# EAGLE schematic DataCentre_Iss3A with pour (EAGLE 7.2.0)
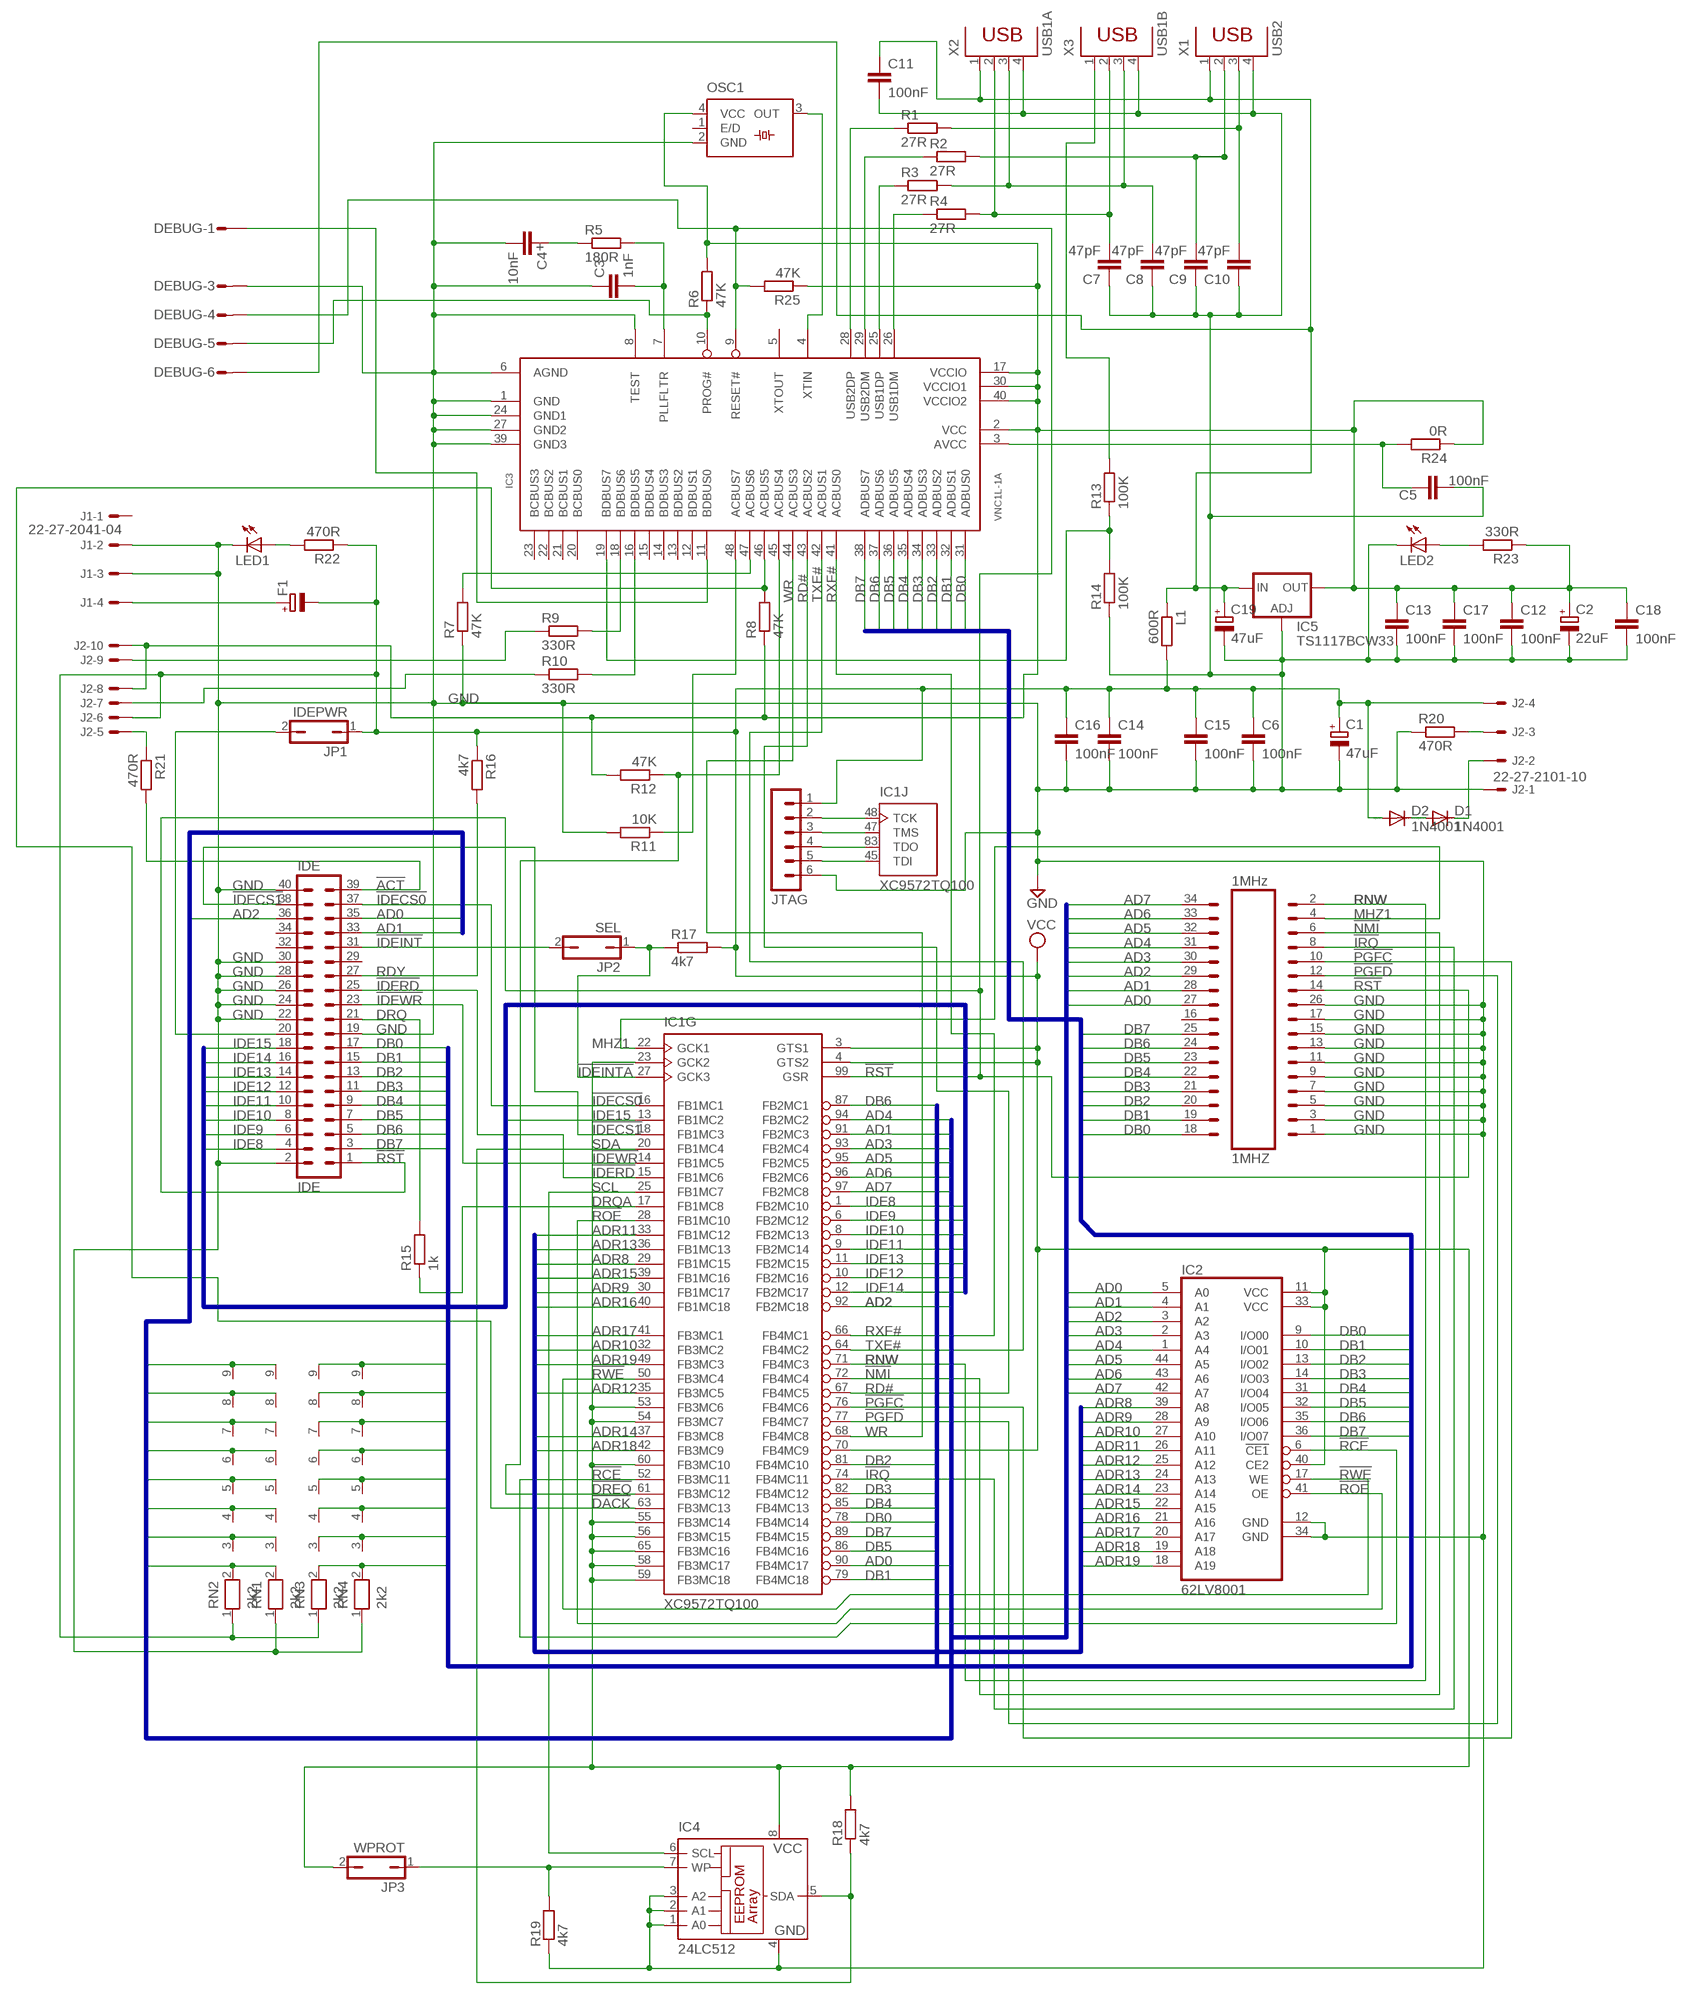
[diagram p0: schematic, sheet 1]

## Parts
C1  47uF  CPOL-EUC  [PANASONIC_C]
C2  22uF  CPOL-EUB  [PANASONIC_B]
C3  1nF  C-EUC1206K  [C1206K]
C4  10nF  C-EUC1206K  [C1206K]
C5  100nF  C-EUC1206K  [C1206K]
C6  100nF  C-EUC1206K  [C1206K]
C7  47pF  C-EUC0603K  [C0603K]
C8  47pF  C-EUC0603K  [C0603K]
C9  47pF  C-EUC0603K  [C0603K]
C10  47pF  C-EUC0603K  [C0603K]
C11  100nF  C-EUC1206K  [C1206K]
C12  100nF  C-EUC1206K  [C1206K]
C13  100nF  C-EUC1206K  [C1206K]
C14  100nF  C-EUC1206K  [C1206K]
C15  100nF  C-EUC1206K  [C1206K]
C16  100nF  C-EUC1206K  [C1206K]
C17  100nF  C-EUC1206K  [C1206K]
C18  100nF  C-EUC0603K  [C0603K]
C19  47uF  CPOL-EUC  [PANASONIC_C]
D1  1N4001  DIODE-DO35-10  [DO35-10]
D2  1N4001  DIODE-DO35-10  [DO35-10]
DEBUG  DF3-06P  [DF3P-06]
F1  CPOL-EU085CS-1R  [085CS_1R]
IC1  XC9572TQ100  [TQ100]
IC2  62LV8001  [TSOPII-Z44]
IC3  VNC1L-1A  [LQFP48]
IC4  24LC512  24LC256SN  [SO-08]
IC5  TS1117BCW33  LD117AS33TR  [SOT223]
IDE  IDE  ML40  [ML40]
J1  22-27-2041-04  [6410-04]
J2  22-27-2101-10  [6410-10]
JP1  IDEPWR  JP1Q  [JP1]
JP2  SEL  JP1Q  [JP1]
JP3  WPROT  JP1Q  [JP1]
JTAG  MA06-1  [MA06-1]
L1  600R  R-EU_R1206  [R1206]
LED1  LEDCHIPLED_0603  [CHIPLED_0603]
LED2  LEDCHIPLED_0603  [CHIPLED_0603]
OSC1  SM77HCSX750  [XTAL-CSX750]
PL1  1MHZ  [ML34]
R1  27R  R-EU_R0603  [R0603]
R2  27R  R-EU_R0603  [R0603]
R3  27R  R-EU_R0603  [R0603]
R4  27R  R-EU_R0603  [R0603]
R5  180R  R-EU_R0603  [R0603]
R6  47K  R-EU_R0603  [R0603]
R7  47K  R-EU_R0603  [R0603]
R8  47K  R-EU_R0603  [R0603]
R9  330R  R-EU_R0603  [R0603]
R10  330R  R-EU_R0603  [R0603]
R11  10K  R-EU_R0603  [R0603]
R12  47K  R-EU_R0603  [R0603]
R13  100K  R-EU_R0603  [R0603]
R14  100K  R-EU_R0603  [R0603]
R15  1k  R-EU_R0603  [R0603]
R16  4k7  R-EU_R0603  [R0603]
R17  4k7  R-EU_R0603  [R0603]
R18  4k7  R-EU_R0603  [R0603]
R19  4k7  R-EU_R0603  [R0603]
R20  470R  R-EU_R0603  [R0603]
R21  470R  R-EU_R0603  [R0603]
R22  470R  R-EU_R0603  [R0603]
R23  330R  R-EU_R0603  [R0603]
R24  0R  R-EU_R0603  [R0603]
R25  47K  R-EU_R0603  [R0603]
RN1  2k2  RN08  [RN-9]
RN2  2k2  RN08  [RN-9]
RN3  2k2  RN08  [RN-9]
RN4  2k2  RN08  [RN-9]
X1  USB2  PN87520  [PN87520]
X2  USB1A  PN87520  [PN87520]
X3  USB1B  PN61729  [PN61729]

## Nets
!ACT: IDE.39 R21.2
!DACK: IC1.63(G:FB3MC13) IC3.46(ACBUS5) R8.2
!DREQ: IC1.61(G:FB3MC12) IC3.45(ACBUS4) R12.1
!IDECS0: IC1.16(G:FB1MC1) IDE.37
!IDECS1: IC1.18(G:FB1MC3) IDE.38
!IDEINT: IDE.31 JP2.2
!IDEINTA: IC1.27(G:GCK3) JP2.1 R17.1
!IDERD: IC1.15(G:FB1MC6) IDE.25
!IDEWR: IC1.14(G:FB1MC5) IDE.23
!IRQ: IC1.74(G:FB4MC11) PL1.8(8_IRQ)
!NMI: IC1.72(G:FB4MC4) PL1.6(6_NMI)
!PGFC: IC1.76(G:FB4MC6) PL1.10(10_FC)
!PGFD: IC1.77(G:FB4MC7) PL1.12(12_FD)
!RCE: IC1.52(G:FB3MC11) IC2.6(!CE1)
!ROE: IC1.28(G:FB1MC10) IC2.41(OE)
!RST: DEBUG.4 IC1.99(G:GSR) IC3.9(RESET#) IDE.1 PL1.14(14_RST) R25.2
!RWE: IC1.50(G:FB3MC4) IC2.17(WE)
AD0: IC1.90(G:FB4MC17) IC2.5(A0) IDE.35 PL1.27(27_A0) RN1.2 RN2.2
AD1: IC1.91(G:FB2MC3) IC2.4(A1) IDE.33 PL1.28(28_A1) RN1.3 RN2.3
AD2: IC1.92(G:FB2MC18) IC2.3(A2) IDE.36 PL1.29(29_A2) RN1.4 RN2.4
AD3: IC1.93(G:FB2MC4) IC2.2(A3) PL1.30(30_A3) RN1.5 RN2.5
AD4: IC1.94(G:FB2MC2) IC2.1(A4) PL1.31(31_A4) RN1.6 RN2.6
AD5: IC1.95(G:FB2MC5) IC2.44(A5) PL1.32(32_A5) RN1.7 RN2.7
AD6: IC1.96(G:FB2MC6) IC2.43(A6) PL1.33(33_A6) RN1.8 RN2.8
AD7: IC1.97(G:FB2MC8) IC2.42(A7) PL1.34(34_A7) RN1.9 RN2.9
ADR8: IC1.29(G:FB1MC15) IC2.39(A8)
ADR9: IC1.30(G:FB1MC17) IC2.28(A9)
ADR10: IC1.32(G:FB3MC2) IC2.27(A10)
ADR11: IC1.33(G:FB1MC12) IC2.26(A11)
ADR12: IC1.35(G:FB3MC5) IC2.25(A12)
ADR13: IC1.36(G:FB1MC13) IC2.24(A13)
ADR14: IC1.37(G:FB3MC8) IC2.23(A14)
ADR15: IC1.39(G:FB1MC16) IC2.22(A15)
ADR16: IC1.40(G:FB1MC18) IC2.21(A16)
ADR17: IC1.41(G:FB3MC1) IC2.20(A17)
ADR18: IC1.42(G:FB3MC9) IC2.19(A18)
ADR19: IC1.49(G:FB3MC3) IC2.18(A19)
DB0: IC1.78(G:FB4MC14) IC2.9(I/O00) IC3.31(ADBUS0) IDE.17 PL1.18(18_D0) RN3.2 RN4.2
DB1: IC1.79(G:FB4MC18) IC2.10(I/O01) IC3.32(ADBUS1) IDE.15 PL1.19(19_D1) RN3.3 RN4.3
DB2: IC1.81(G:FB4MC10) IC2.13(I/O02) IC3.33(ADBUS2) IDE.13 PL1.20(20_D2) RN3.4 RN4.4
DB3: IC1.82(G:FB4MC12) IC2.14(I/O03) IC3.34(ADBUS3) IDE.11 PL1.21(21_D3) RN3.5 RN4.5
DB4: IC1.85(G:FB4MC13) IC2.31(I/O04) IC3.35(ADBUS4) IDE.9 PL1.22(22_D4) RN3.6 RN4.6
DB5: IC1.86(G:FB4MC16) IC2.32(I/O05) IC3.36(ADBUS5) IDE.7 PL1.23(23_D5) RN3.7 RN4.7
DB6: IC1.87(G:FB2MC1) IC2.35(I/O06) IC3.37(ADBUS6) IDE.5 PL1.24(24_D6) RN3.8 RN4.8
DB7: IC1.89(G:FB4MC15) IC2.36(I/O07) IC3.38(ADBUS7) IDE.3 PL1.25(25_D7) RN3.9 RN4.9
DRQ: IDE.21 R15.2
DRQA: IC1.17(G:FB1MC8) R15.1
GND [Power]: C1.- C2.- C3.1 C4.2 C5.2 C6.2 C7.1 C8.1 C9.1 C10.1 C11.2 C12.2 C13.2 C14.2 C15.2 C16.2 C17.2 C18.2 C19.- DEBUG.3 IC2.12(GND) IC2.34(GND) IC3.1(GND) IC3.6(AGND) IC3.8(TEST) IC3.24(GND1) IC3.27(GND2) IC3.39(GND3) IC4.1(A0) IC4.2(A1) IC4.3(A2) IC4.4(GND) IC5.1(ADJ) IDE.2 IDE.19 IDE.22 IDE.24 IDE.26 IDE.28 IDE.30 IDE.40 J1.2 J1.3 J2.1 JTAG.6 LED1.C LED2.C OSC1.2(GND) PL1.1(1_GND) PL1.3(3_GND) PL1.5(5_GND) PL1.7(7_GND) PL1.9(9_GND) PL1.11(11_GND) PL1.13(13_GND) PL1.15(15_GND) PL1.17(17_GND) PL1.26(26_GND) R7.1 R11.2 R14.1 R19.1 R20.1 RN1.1 RN4.1 X1.4 X2.4 X3.4
IDE8: IC1.1(G:FB2MC10) IDE.4
IDE9: IC1.6(G:FB2MC12) IDE.6
IDE10: IC1.8(G:FB2MC13) IDE.8
IDE11: IC1.9(G:FB2MC14) IDE.10
IDE12: IC1.10(G:FB2MC16) IDE.12
IDE13: IC1.11(G:FB2MC15) IDE.14
IDE14: IC1.12(G:FB2MC17) IDE.16
IDE15: IC1.13(G:FB1MC2) IDE.18
MHZ1: IC1.22(G:GCK1) PL1.4(4_1MHZ)
N$1: IDE.20 JP1.2
N$2 [Power]: F1.+ J1.4
N$3: IC1.48(J:TCK) JTAG.2
N$4: IC1.47(J:TMS) JTAG.3
N$5: IC1.83(J:TDO) JTAG.4
N$6: IC1.45(J:TDI) JTAG.5
N$7: J2.5 R21.1
N$8: IC3.4(XTIN) OSC1.3(OUT)
N$9: LED2.A R23.2
N$10: C3.2 IC3.7(PLLFLTR) R5.2
N$11: C4.1 R5.1
N$12: DEBUG.5 IC3.10(PROG#) R6.1
N$13: J2.7 R10.1
N$14: IC3.26(USB1DM) R4.1
N$15: J2.3 R20.2
N$16: IC3.25(USB1DP) R3.1
N$17: D1.A D2.C
N$18: D1.C J2.2
N$19: IC3.29(USB2DM) R2.1
N$20: IC3.28(USB2DP) R1.1
N$21: C7.2 R4.2 X2.2 X3.2
N$22: C8.2 R3.2 X2.3 X3.3
N$23: C9.2 R2.2 X1.2
N$24: C10.2 R1.2 X1.3
N$25: J2.9 R9.1
N$26: IC3.16(BDBUS5) R10.2
N$28: IC3.47(ACBUS6) R7.2
N$29: IC3.18(BDBUS6) R9.2
N$31: R13.2 X3.1
N$36: IC3.48(ACBUS7) R11.1
N$37: LED1.A R22.2
N$43: DEBUG.1 IC3.11(BDBUS0)
N$50: C5.1 IC3.3(AVCC) R24.2
RD#: IC1.67(G:FB4MC5) IC3.43(ACBUS2)
RDY: IDE.27 R16.2
RNW: IC1.71(G:FB4MC3) PL1.2(2_RW)
RXF#: IC1.66(G:FB4MC1) IC3.41(ACBUS0)
SCL: IC1.25(G:FB1MC7) IC4.6(SCL)
SDA: IC1.20(G:FB1MC4) IC4.5(SDA) R18.1
SWP: IC4.7(WP) JP3.1 R19.2
TXE#: IC1.64(G:FB4MC2) IC3.42(ACBUS1)
UBVCC: IC3.19(BDBUS7) R13.1 R14.2
VCC [Power]: C1.+ C6.1 C14.1 C15.1 C16.1 D2.A F1.- IC1.3(G:GTS1) IC1.4(G:GTS2) IC1.23(G:GCK2) IC1.53(G:FB3MC6) IC1.54(G:FB3MC7) IC1.55(G:FB3MC14) IC1.56(G:FB3MC15) IC1.58(G:FB3MC17) IC1.59(G:FB3MC18) IC1.60(G:FB3MC10) IC1.65(G:FB3MC16) IC1.70(G:FB4MC9) IC2.11(VCC) IC2.33(VCC) IC2.40(CE2) IC4.8(VCC) J2.4 J2.6 JP1.1 JP3.2 JTAG.1 L1.2 R16.1 R17.2 R18.2 R22.1 RN2.1 RN3.1
VCC3V3 [Power]: C2.+ C12.1 C13.1 C17.1 C18.1 IC3.2(VCC) IC3.17(VCCIO) IC3.30(VCCIO1) IC3.40(VCCIO2) IC5.4(OUT) J2.8 J2.10 OSC1.4(VCC) R6.2 R8.1 R12.2 R23.1 R24.1 R25.1
VCC_RF [Power]: C11.1 C19.+ DEBUG.6 IC5.3(IN) L1.1 X1.1 X2.1
WR: IC1.68(G:FB4MC8) IC3.44(ACBUS3)
Unconnected: IC3.5(XTOUT) IC3.12(BDBUS1) IC3.13(BDBUS2) IC3.14(BDBUS3) IC3.15(BDBUS4) IC3.20(BCBUS0) IC3.21(BCBUS1) IC3.22(BCBUS2) IC3.23(BCBUS3) IDE.29 IDE.32 IDE.34 J1.1 OSC1.1(E/D) PL1.16(16_ANALOG)

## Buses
ADR[8..19]
DB[0..7]
AD[0..7]
IDE[8..15]

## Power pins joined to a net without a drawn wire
GND: IC1.21(P:GND) IC1.31(P:GND) IC1.44(P:GND) IC1.62(P:GND) IC1.69(P:GND) IC1.75(P:GND) IC1.84(P:GND) IC1.100(P:GND)
VCC: IC1.5(P:VCC) IC1.26(P:VCC) IC1.38(P:VCC) IC1.51(P:VCC) IC1.57(P:VCC) IC1.88(P:VCC) IC1.98(P:VCC)

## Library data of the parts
C1 C2 C19 F1 = resistor:CPOL-EU: POLARIZED CAPACITOR, European symbol
C3 C5-C18 = resistor:C-EU: CAPACITOR, European symbol
C4 = rcl:C-EU: CAPACITOR, European symbol; POL: +
D1 D2 = diode:DIODE-: DIODE
DEBUG = con-hirose-df3:DF3-06: Single row connector 2mm 6 way
IC1 = XILINX:XC9572TQ100
IC2 = memory-sram:62LV8001
IC3 = ftdichip-1:VNC1L
IC4 = microchip:24*: Serial EEPROM I2C; MF: MICROCHIP; MPN: 24LC256-I/SN; OC_FARNELL: 9757996; OC_NEWARK: 27C9144
IC5 = v-reg:LD117A?*: Low drop fixed and adjustable positive voltage regulators 1 A Source: http://www.st.com/stonline/products/literature/ds/7194/ld1117axx.pdf
IDE = con-harting-ml:ML40: HARTING; OC_FARNELL: unknown; OC_NEWARK: unknown
J1 = con-molex:22-?-04: CONNECTOR wire to board 2.54 mm (.1 inch) pitch header; OC_FARNELL: unknown; OC_NEWARK: unknown
J2 = con-molex:22-?-10: CONNECTOR wire to board 2.54 mm (.1 inch) pitch header; OC_FARNELL: unknown; OC_NEWARK: unknown
JP1-JP3 = jumper:JP1Q: JUMPER
JTAG = con-lstb:MA06-1: PIN HEADER; OC_FARNELL: unknown; OC_NEWARK: unknown
L1 R1-R25 = resistor:R-EU_: RESISTOR, European symbol
LED1 LED2 = led:LED: LED
OSC1 = jt-crystals:SM77H: 3.3V CMOS Clock Oscillator Source: www.pletronics.com .. sm77h%203.3v.pdf
PL1 = BBC:1MHZ: 1MHz Bus
RN1-RN4 = resistor-net:RN08: RESISTOR NETWORK; OC_FARNELL: unknown; OC_NEWARK: unknown
X1 X2 = con-berg:PN87520: BERG USB connector; OC_FARNELL: unknown; OC_NEWARK: unknown
X3 = con-berg:PN61729: BERG USB connector; OC_FARNELL: unknown; OC_NEWARK: unknown

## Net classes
0 Signal: width 0.254 mm
1 Power: width 0.305 mm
